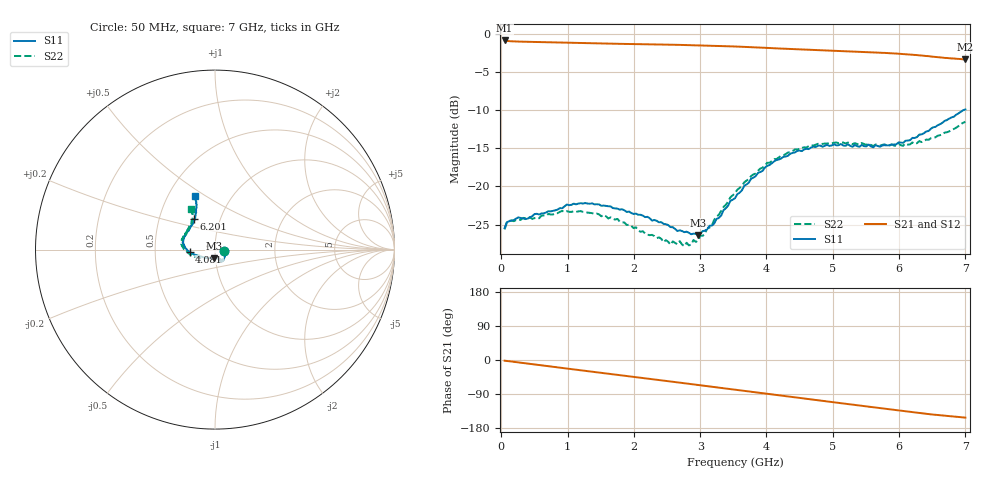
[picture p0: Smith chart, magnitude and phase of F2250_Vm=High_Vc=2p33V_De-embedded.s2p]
! Integrated Device Technology
! Corporate Headquarters
! 6024 Silver Creek Valley Road
! San Jose, CA 95138  USA
! Phone:  1-408-284-8200
! Toll Free:  1-800-223-1366
! Webpage:  http://www.idt.com/
! Timing and RF Division
! 515 Groton Road, Suite 102
! Westford, MA 01886-6024
! Device:  F2250
! Description: Voltage Variable RF Attenuator
! Frequency:  50.0 -  6000.00 MHz
! Package:  3x3 mm Thin QFN Plastic Package: 16 pin
! Ports:  2 RF, 3 DC
!  Pin  1  = GND
!  Pin  2  = NC
!  Pin  3  = RF1  = Port 1
!  Pin  4  = NC
!  Pin  5  = GND
!  Pin  6  = GND
!  Pin  7  = GND
!  Pin  8  = GND
!  Pin  9  = NC
!  Pin 10  = RF2  = Port 2
!  Pin 11  = NC
!  Pin 12  = GND
!  Pin 13  = GND
!  Pin 14  = VCNTRL
!  Pin 15  = VDD
!  Pin 16  = VMODE
! Vcntrl:  2.330 Volts
! Vmode:  +3.300 Volts
! Vdd:  +3.30  Volts
! Current:  1.316 mA
! Data:  The device was measured on a the F2250 evaluation board which has
!  individual transmission lines to the RF pins.  Data was collected
!  using a calibrated network analyzer.  The evaluation board was
!  de-embedded using a TRL calibration technique.
!  The reference plane is the edge of the package pin.
! Misc:  SN 10
!  Action Tracker AT0258
! Date Measured:  2014-11-26
! Date:  2015-10-15  MJV
! Note:
!  Integrated Device Technology supplies this data as a sample of measured
!  data at the package pin for this product.  Your particular data for this
!  product may vary.
!  Data was taken at 25 degrees C.
!  Integrated Device Technology reserves the right to change this data at anytime.
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# GHz S dB R 50
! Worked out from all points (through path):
!   201 points, 50 MHz to 7 GHz, reference 50 ohm
!   highest |S21| = -0.90 dB at 50 MHz (marker M1); lowest = -3.4 dB at 7 GHz (marker M2)
!   group delay of S21, straight-line fit = 61.2 ps
!   lowest |S11| = -26.4 dB at 2.969 GHz (marker M3), VSWR 1.10, Z = 49.2 - j4.72 ohm
!   |S11| at or under -10 dB: start of sweep to 6.977 GHz
!   |S22| runs from -27.8 to -11.5 dB; largest |S21 - S12| = 0.0019
!   S11 on the Smith chart (normalised r, x): 50 MHz: 1.11, -0.02; 4.081 GHz: 0.75, -0.02; 6.201 GHz: 0.75, +0.27; 7 GHz: 0.68, +0.45
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0.05  -25.47 -10.5  -0.90 -1.8  -0.90 -1.8  -25.64 -10.8
0.1195  -24.57 -10.1  -1.00 -3.2  -1.00 -3.2  -24.52 -8.8
0.57125  -23.68 -30.9  -1.11 -13.3  -1.11 -13.3  -24.17 -31.2
0.91875  -22.87 -49.6  -1.18 -21.0  -1.18 -21.1  -23.21 -50.7
1.2315  -22.25 -57.3  -1.25 -27.9  -1.25 -27.9  -23.33 -61.2
1.75275  -22.92 -64.3  -1.34 -39.1  -1.34 -39.1  -24.26 -67.6
2.37825  -24.70 -64.0  -1.43 -52.8  -1.43 -52.8  -26.67 -67.1
2.552  -25.33 -68.8  -1.46 -56.7  -1.46 -56.7  -27.63 -73.5
2.691  -25.75 -76.8  -1.48 -59.8  -1.48 -59.8  -27.17 -81.2
2.7605  -26.00 -79.0  -1.50 -61.3  -1.50 -61.3  -27.83 -85.6
2.969  -26.35 -96.8  -1.54 -66.0  -1.54 -66.0  -27.09 -104.9
3.1775  -25.14 -119.8  -1.58 -70.7  -1.58 -70.7  -25.10 -126.5
3.525  -21.55 -152.0  -1.69 -78.5  -1.69 -78.6  -20.90 -148.5
3.76825  -18.99 -164.2  -1.78 -84.0  -1.78 -84.1  -18.65 -159.5
4.081  -16.98 -175.3  -1.91 -91.0  -1.91 -91.0  -16.68 -171.3
4.4285  -15.57 176.3  -2.04 -98.6  -2.05 -98.7  -15.17 178.8
4.7065  -14.79 169.4  -2.14 -104.8  -2.14 -104.8  -14.66 173.0
5.054  -14.63 161.2  -2.27 -112.5  -2.27 -112.5  -14.26 166.0
5.85325  -14.61 135.3  -2.57 -130.0  -2.57 -130.1  -14.67 147.3
6.20075  -13.65 123.8  -2.78 -137.7  -2.78 -137.8  -14.25 138.3
6.54825  -12.22 115.8  -3.05 -144.7  -3.05 -144.9  -13.58 126.9
7  -9.94 110.9  -3.38 -152.1  -3.39 -152.2  -11.55 120.7
